
DATA_BLOCK DB3497
TITLE=
VERSION : 0.1

STRUCT
   CM_ID : STRING  [8 ] := '=PRM'; //COMPOSITE MACHINE
   STATION_ID : STRING  [8 ] := '++OP10'; //STATION - TRATTO - ZONE
   ELEMENT_ID : STRING  [8 ] := '+82MO21'; //ELEMENT
   DB_ID : INT := 0 ; //DB SIZE OR TYPE
   PART_STYLE : STRING  [12 ]; //PART STYLE ON LAST STATION
   ACT_CYCLE_TIME : INT ; //ACTUAL CYCLE TIME FOR THIS STYLE
   COUNT_GOOD : INT ; //COUNTER GOOD PIECES
   COUNT_SCRAP : INT ; //COUNTER SCRAP PIECES
   SPARE_00 : ARRAY  [0 .. 15 ] OF //SPARE INTEGER
   INT ;
   SPARE_01 : ARRAY  [0 .. 17 ] OF //SPARE INTEGER
   INT ;
   CODE_EVENT : ARRAY  [0 .. 7 ] OF //CODE EVENT - EXTENDED FAULT CODE DIAGNOSTIC
   INT ;
   EVENT : STRUCT
E0000 : BOOL ; //+82MO21-B51_1; MS. G82_MO21_B51_1 ALLARME;58
E0001 : BOOL ; //+82MO21-B51_1; MS. G82_MO21_B51_1_PRE ALLARME;58
E0002 : BOOL ; //+82MO21-B51_1; ME. G82_MO21_B51_1 ALLARME;01
E0003 : BOOL ; //+82MO21-B51_1; ME. G82_MO21_B51_1_PRE ALLARME;01
E0004 : BOOL ; //+82MO21-B51_1; ME. G82_MO21_B51_1 PLAUSIBILITA;2
E0005 : BOOL ; //+82MO21-B51_2; MS. G82_MO21_B51_2 ALLARME;58
E0006 : BOOL ; //+82MO21-B51_2; MS. G82_MO21_B51_2_PRE ALLARME;58
E0007 : BOOL ; //+82MO21-B51_2; ME. G82_MO21_B51_2 ALLARME;01
E0008 : BOOL ; //+82MO21-B51_2; ME. G82_MO21_B51_2_PRE ALLARME;01
E0009 : BOOL ; //+82MO21-B51_2; ME. G82_MO21_B51_2 PLAUSIBILITA;2
E0010 : BOOL ;
E0011 : BOOL ;
E0012 : BOOL ;
E0013 : BOOL ;
E0014 : BOOL ;
E0015 : BOOL ;
E0016 : BOOL ;
E0017 : BOOL ;
E0018 : BOOL ;
E0019 : BOOL ;
E0020 : BOOL ;
E0021 : BOOL ;
E0022 : BOOL ;
E0023 : BOOL ;
E0024 : BOOL ;
E0025 : BOOL ;
E0026 : BOOL ;
E0027 : BOOL ;
E0028 : BOOL ;
E0029 : BOOL ;
E0030 : BOOL ;
E0031 : BOOL ;
E0032 : BOOL ;
E0033 : BOOL ;
E0034 : BOOL ;
E0035 : BOOL ;
E0036 : BOOL ;
E0037 : BOOL ;
E0038 : BOOL ;
E0039 : BOOL ;
E0040 : BOOL ;
E0041 : BOOL ;
E0042 : BOOL ;
E0043 : BOOL ;
E0044 : BOOL ;
E0045 : BOOL ;
E0046 : BOOL ;
E0047 : BOOL ;
E0048 : BOOL ;
E0049 : BOOL ;
E0050 : BOOL ;
E0051 : BOOL ;
E0052 : BOOL ;
E0053 : BOOL ;
E0054 : BOOL ;
E0055 : BOOL ;
E0056 : BOOL ;
E0057 : BOOL ;
E0058 : BOOL ;
E0059 : BOOL ;
E0060 : BOOL ;
E0061 : BOOL ;
E0062 : BOOL ;
E0063 : BOOL ;
END_STRUCT;
END_STRUCT;
BEGIN
CM_ID := '=PRM';
STATION_ID := '++OP10';
ELEMENT_ID := '+82MO21';
DB_ID := 1 ;
PART_STYLE := '';
ACT_CYCLE_TIME := 0;
COUNT_GOOD := 0;
COUNT_SCRAP := 0;
SPARE_00[0] := 0;
SPARE_00[1] := 0;
SPARE_00[2] := 0;
SPARE_00[3] := 0;
SPARE_00[4] := 0;
SPARE_00[5] := 0;
SPARE_00[6] := 0;
SPARE_00[7] := 0;
SPARE_00[8] := 0;
SPARE_00[9] := 0;
SPARE_00[10] := 0;
SPARE_00[11] := 0;
SPARE_00[12] := 0;
SPARE_00[13] := 0;
SPARE_00[14] := 0;
SPARE_00[15] := 0;
SPARE_01[0] := 0;
SPARE_01[1] := 0;
SPARE_01[2] := 0;
SPARE_01[3] := 0;
SPARE_01[4] := 0;
SPARE_01[5] := 0;
SPARE_01[6] := 0;
SPARE_01[7] := 0;
SPARE_01[8] := 0;
SPARE_01[9] := 0;
SPARE_01[10] := 0;
SPARE_01[11] := 0;
SPARE_01[12] := 0;
SPARE_01[13] := 0;
SPARE_01[14] := 0;
SPARE_01[15] := 0;
SPARE_01[16] := 0;
SPARE_01[17] := 0;
CODE_EVENT[0] := 0;
CODE_EVENT[1] := 0;
CODE_EVENT[2] := 0;
CODE_EVENT[3] := 0;
CODE_EVENT[4] := 0;
CODE_EVENT[5] := 0;
CODE_EVENT[6] := 0;
CODE_EVENT[7] := 0;
EVENT.E0000 := FALSE;
EVENT.E0001 := FALSE;
EVENT.E0002 := FALSE;
EVENT.E0003 := FALSE;
EVENT.E0004 := FALSE;
EVENT.E0005 := FALSE;
EVENT.E0006 := FALSE;
EVENT.E0007 := FALSE;
EVENT.E0008 := FALSE;
EVENT.E0009 := FALSE;
EVENT.E0010 := FALSE;
EVENT.E0011 := FALSE;
EVENT.E0012 := FALSE;
EVENT.E0013 := FALSE;
EVENT.E0014 := FALSE;
EVENT.E0015 := FALSE;
EVENT.E0016 := FALSE;
EVENT.E0017 := FALSE;
EVENT.E0018 := FALSE;
EVENT.E0019 := FALSE;
EVENT.E0020 := FALSE;
EVENT.E0021 := FALSE;
EVENT.E0022 := FALSE;
EVENT.E0023 := FALSE;
EVENT.E0024 := FALSE;
EVENT.E0025 := FALSE;
EVENT.E0026 := FALSE;
EVENT.E0027 := FALSE;
EVENT.E0028 := FALSE;
EVENT.E0029 := FALSE;
EVENT.E0030 := FALSE;
EVENT.E0031 := FALSE;
EVENT.E0032 := FALSE;
EVENT.E0033 := FALSE;
EVENT.E0034 := FALSE;
EVENT.E0035 := FALSE;
EVENT.E0036 := FALSE;
EVENT.E0037 := FALSE;
EVENT.E0038 := FALSE;
EVENT.E0039 := FALSE;
EVENT.E0040 := FALSE;
EVENT.E0041 := FALSE;
EVENT.E0042 := FALSE;
EVENT.E0043 := FALSE;
EVENT.E0044 := FALSE;
EVENT.E0045 := FALSE;
EVENT.E0046 := FALSE;
EVENT.E0047 := FALSE;
EVENT.E0048 := FALSE;
EVENT.E0049 := FALSE;
EVENT.E0050 := FALSE;
EVENT.E0051 := FALSE;
EVENT.E0052 := FALSE;
EVENT.E0053 := FALSE;
EVENT.E0054 := FALSE;
EVENT.E0055 := FALSE;
EVENT.E0056 := FALSE;
EVENT.E0057 := FALSE;
EVENT.E0058 := FALSE;
EVENT.E0059 := FALSE;
EVENT.E0060 := FALSE;
EVENT.E0061 := FALSE;
EVENT.E0062 := FALSE;
EVENT.E0063 := FALSE;
END_DATA_BLOCK
